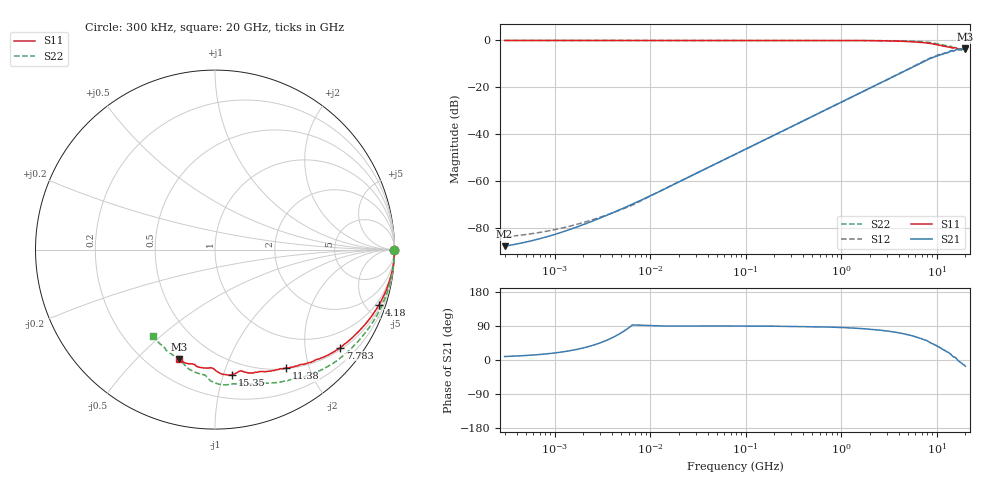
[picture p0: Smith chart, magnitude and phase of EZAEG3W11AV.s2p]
!*** S-Parameter ***
!Copyright (C)  Panasonic Industry
!ESD Suppressor, High Withstanding Type
!Parts No.  EZAEG3W11AV
! Size : 1608mm
# hz S ma R 50
! 2 Port Network Data from SP1.SP block
! freq  magS11  angS11  magS21  angS21  magS12  angS12  magS22  angS22
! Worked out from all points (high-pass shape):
!   966 points, 300 kHz to 20 GHz, reference 50 ohm
!   highest |S21| = -3.17 dB at 20 GHz (marker M1); lowest = -87.9 dB at 300 kHz (marker M2)
!   |S21| within 3 dB of the highest: 10.73908 GHz to 10.79008 GHz (50.99 MHz wide, 0.474 % of centre); 10.88 GHz to end of sweep
!   lowest |S11| = -3.8 dB at 20 GHz (marker M3), VSWR 4.60, Z = 16.2 - j33.6 ohm
!   |S11| at or under -10 dB: nowhere
!   |S22| runs from -4.6 to 0.0 dB; largest |S21 - S12| = 0.042
!   S11 on the Smith chart (normalised r, x): 300 kHz: open; 4.18 GHz: 0.69, -5.99; 7.783 GHz: 0.55, -2.80; 11.38 GHz: 0.51, -1.65; 15.35 GHz: 0.39, -1.07; 20 GHz: 0.32, -0.67
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300000  1 -0.0  4.019e-05 9.2  6.36e-05 25.2  0.9998 -0.0
1221753  1 -0.0  8.128e-05 21.5  9.887e-05 34.7  0.9998 -0.0
1610483  1 -0.0  9.861e-05 26.7  0.0001137 38.7  0.9998 -0.0
1913988  1 -0.0  0.0001121 30.7  0.0001254 41.9  0.9998 -0.0
3364215  0.9999 -0.0  0.0001768 50.1  0.0001808 56.9  0.9998 -0.0
6263581  1 -0.0  0.0003061 88.7  0.0002918 86.9  1 -0.0
1.221117e7  0.9999 -0.0  0.0005767 89.9  0.0005786 90.6  1 -0.0
7.790674e7  0.9998 -0.3  0.003703 89.7  0.003695 89.7  1 -0.3
4.970419e8  0.9994 -2.0  0.02362 88.0  0.02355 88.1  0.9997 -2.0
1.449732e9  0.9954 -6.1  0.06901 83.8  0.06889 84.1  0.9976 -6.2
2.219453e9  0.9893 -9.6  0.1056 80.2  0.1058 80.6  0.9944 -9.6
3.171107e9  0.9785 -13.9  0.1512 75.8  0.1521 76.4  0.9883 -14.2
4.180072e9  0.9636 -18.7  0.1995 71.0  0.2017 71.2  0.9794 -19.2
5.904048e9  0.9301 -27.5  0.2828 61.8  0.289 62.3  0.9573 -28.8
7.782564e9  0.8857 -38.1  0.3754 51.5  0.3833 51.0  0.9227 -40.9
9.249234e9  0.8398 -46.5  0.4363 42.2  0.4448 41.6  0.8809 -51.1
1.137851e10  0.7704 -59.0  0.5091 29.1  0.518 28.5  0.8086 -66.6
1.383777e10  0.7171 -73.6  0.5822 16.6  0.5908 13.8  0.7558 -85.1
1.534815e10  0.7023 -82.3  0.603 7.8  0.6017 5.4  0.6961 -97.6
1.663597e10  0.6611 -91.1  0.6444 -0.4  0.6385 -3.4  0.6438 -107.1
1.910005e10  0.6532 -103.6  0.6693 -12.1  0.6582 -14.5  0.6073 -120.6
2e10  0.6426 -108.3  0.6942 -16.5  0.6756 -18.6  0.5914 -125.4
